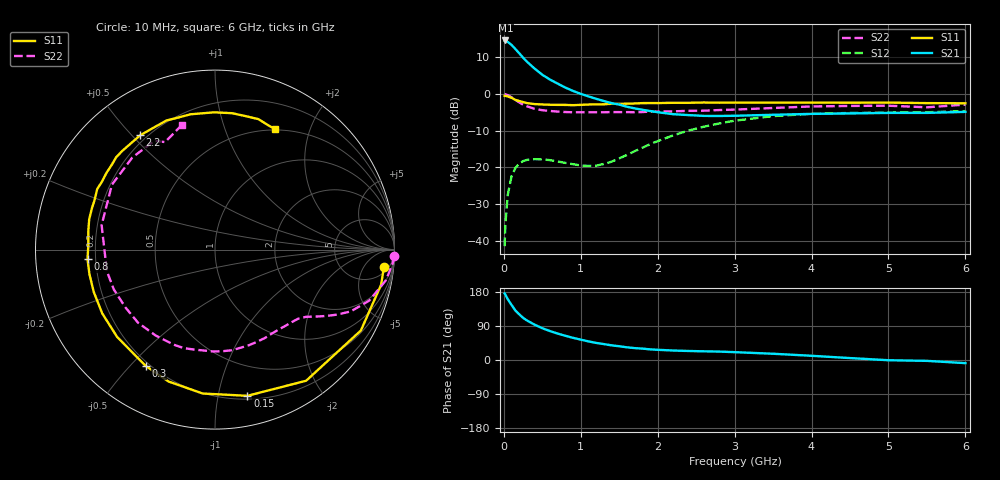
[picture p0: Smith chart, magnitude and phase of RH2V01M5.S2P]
! SIEMENS Small Signal Semiconductors
! BFR106
! Si NPN RF Bipolar Junction Transistor in SOT23
! VCE = 2 V  IC = 1.5 mA
! Common Emitter S-Parameters:  August  1996
# GHz  S  MA  R  50
!  f  S11  S21  S12  S22
! GHz  MAG  ANG  MAG  ANG  MAG  ANG  MAG  ANG
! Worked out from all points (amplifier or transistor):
!   36 points, 10 MHz to 6 GHz, reference 50 ohm
!   highest |S21| = 14.6 dB at 20 MHz (marker M1)
!   |S21| within 3 dB of that: start of sweep to 178.9 MHz
!   unconditionally stable (mu >= 1): 808.2 MHz to end of sweep
!   at 250 MHz: K = 0.29, MSG = 14.1 dB, |S12| = -18.3 dB
!   at 1.4 GHz: K = 1.36, MAG = 4.4 dB, |S12| = -18.5 dB
!   at 6 GHz: K = 1.02, MAG = -1.0 dB, |S12| = -4.6 dB
!   S11 on the Smith chart (normalised r, x): 10 MHz: 8, -15; 150 MHz: 0.23, -1.22; 300 MHz: 0.18, -0.55; 800 MHz: 0.17, -0.04; 2.2 GHz: 0.17, +0.53; 6 GHz: 0.49, +1.51
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0.01  0.9461 -5.9  5.384 175.6  0.0084 87.3  0.9977 -2.1
0.02  0.9461 -11.9  5.399 172.6  0.0167 83.1  0.9933 -4.2
0.05  0.9294 -29.0  5.171 160.8  0.0417 73.4  0.9689 -10.0
0.1  0.8898 -55.2  4.693 145.3  0.0754 60.0  0.9051 -18.3
0.15  0.8344 -77.5  4.129 130.7  0.0981 48.3  0.8322 -24.4
0.2  0.8048 -94.9  3.613 120.6  0.1126 40.6  0.7715 -28.0
0.25  0.7791 -109.4  3.146 111.2  0.1215 33.6  0.7184 -31.0
0.3  0.7543 -120.8  2.773 104.4  0.1265 29.4  0.6824 -33.1
0.4  0.731 -138.2  2.228 93.2  0.1295 23.1  0.6298 -36.5
0.5  0.7219 -150.5  1.836 83.9  0.1287 19.3  0.6025 -39.7
0.6  0.7155 -160.8  1.578 76.3  0.1255 17.5  0.5884 -43.4
0.8  0.7122 -175.7  1.227 63.9  0.1152 19.0  0.5695 -51.5
1.1  0.7211 166.4  0.931 49.1  0.1045 32.3  0.5647 -65.5
1.6  0.7405 144.7  0.672 33.5  0.1478 60.3  0.5677 -91.1
2.2  0.7612 123.2  0.532 25.0  0.2731 61.8  0.5817 -124.5
2.8  0.7637 105.3  0.503 22.2  0.3976 49.2  0.6059 -158.5
3.5  0.7649 90.4  0.522 16.5  0.5007 32.3  0.6463 167.8
4  0.7659 82.9  0.537 11.1  0.538 21.2  0.6787 147.8
4.5  0.7631 76.9  0.545 5.1  0.5527 11.9  0.6895 131.9
5  0.7659 71.6  0.554 -0.6  0.5594 4.5  0.6941 119.2
5.5  0.7534 66.7  0.554 -2.3  0.565 1.0  0.6605 114.9
6  0.7495 63.3  0.572 -8.3  0.5863 -6.4  0.7189 104.8
